(* Logix 5000 AddOnInstructionDefinition export; software revision 16.04 *)

TYPE AKD_Status :   // All connections to the drive ethernet module are established and data is successfully transferring.
STRUCT
   Profile_In_Progress : BOOL;   // Profile Move In Progress
   Block_In_Execution : BOOL;   // Block In Execution
   On_Target_Position : BOOL;   // On Target Position (1=Current Position Equals Last Target Position)
   General_Fault : BOOL;   // General Fault
   Current_Direction : BOOL;   // Current Motor Direction (0=Reverse, 1=Forward)
   Home_Level : BOOL;   // Level of Home Input
   Reg_Level : BOOL;   // Level of Registration Input
   Enable : BOOL;   // State of Enable Output
   Fault_Input_Fault : BOOL;   // Fault Input Active
   Fwd_Limit : BOOL;   // Forward Input Active
   Rev_Limit : BOOL;   // Reverse Input Active
   Positive_Limit : BOOL;   // Positive Software Limit Exceeded
   Negative_Limit : BOOL;   // Negative Software Limit Exceeded
   FE_Fault : BOOL;   // Following Error Fault
   Block_Fault : BOOL;   // Block Execution Fault
   Load_Complete : BOOL;   // Command Message Successfully Loaded
END_STRUCT
END_TYPE

TYPE AKD_Axis :   // Axis Data:
STRUCT
   Control : AKD_Control;   // Control bits to send to the drive
   Status : AKD_Status;   // Status bits received from the drive
   Input : AB:ETHERNET_MODULE_SINT_64Bytes:I:0;   // Data from the drive
   Output : AB:ETHERNET_MODULE_SINT_64Bytes:O:0;   // Data to the drive
   ResponseMsgType : SINT;   // Response type contained in latest IO response from drive. Used to check for errors
   CommandTimeout : INT;   // Time to allow for command response from drive. Dependent on scan rate and communicaiton rate
   PositionFeedback : DINT;   // Actual Position Value
   VelocityFeedback : DINT;   // Actual Velocity Value
END_STRUCT
END_TYPE

TYPE AKD_Control :   // Send Explicit Message
STRUCT
   Load_Data_Start_Profile : BOOL;   // Load Command Data / Start Profile Move
   Start_Block : BOOL;   // Execute Command block or block chain
   Incremental : BOOL;   // Incremental Position (0=Absolute, 1=Incremental)
   Direction : BOOL;   // Direction in Velocity Mode (0=Reverse, 1=Forward)
   Smooth_Stop : BOOL;   // Smooth / Controlled Stop w/ Deceleration
   Hard_Stop : BOOL;   // Hard / Immediate Stop
   Reg_Arm : BOOL;   // Arm the Registration Input
   Enable : BOOL;   // Enable Output
END_STRUCT
END_TYPE

ADD_ON_INSTRUCTION AKD_Enable   (* revision 2.0, ExecutePrescan, ExecuteEnableInFalse *)
// Enables Drive
VAR_OUTPUT
   DN : BOOL; {visible}   // Command Successful
   ER : BOOL; {visible}   // Error
END_VAR
VAR_IN_OUT
   Axis : AKD_Axis; {required}
END_VAR
VAR
   Command_Timeout : TIMER;   // Timeout Timer
   Transition : BOOL;   // Marker to transition enable bit if required.
   Transition_Complete : BOOL;   // Flag to indicate that no further transistion is required.
END_VAR

ROUTINE EnableInFalse   (* ladder *)
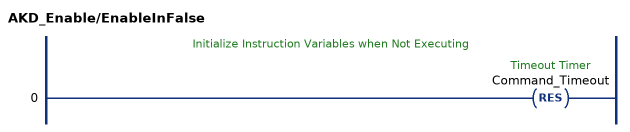
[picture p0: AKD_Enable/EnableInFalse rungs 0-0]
   // Initialize Instruction Variables when Not Executing
   0: RES(Command_Timeout);
END_ROUTINE

ROUTINE Logic   (* ladder *)
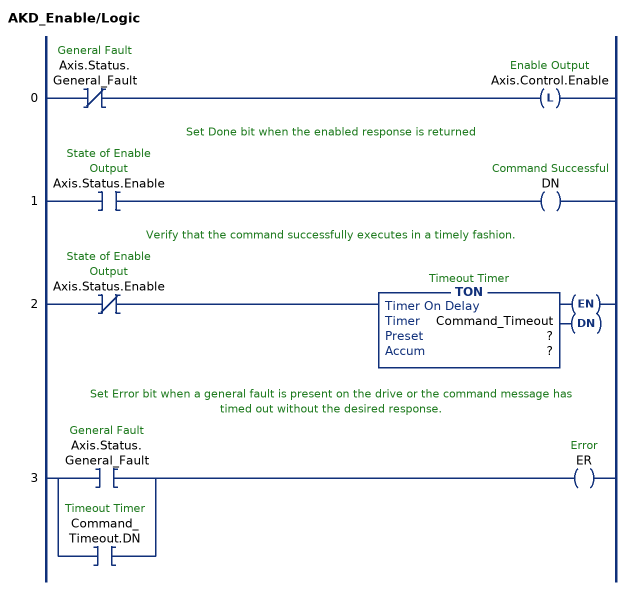
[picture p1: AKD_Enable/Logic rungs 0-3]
   0: XIO(Axis.Status.General_Fault)OTL(Axis.Control.Enable);
   // Set Done bit when the enabled response is returned
   1: XIC(Axis.Status.Enable)OTE(DN);
   // Verify that the command successfully executes in a timely fashion.
   2: XIO(Axis.Status.Enable)TON(Command_Timeout,?,?);
   // Set Error bit when a general fault is present on the drive or the command message has timed out without the desired response.
   3: [XIC(Axis.Status.General_Fault) ,XIC(Command_Timeout.DN) ]OTE(ER);
END_ROUTINE

ROUTINE Prescan   (* ladder *)
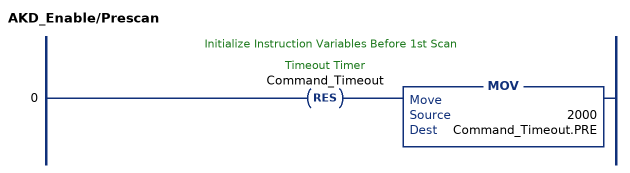
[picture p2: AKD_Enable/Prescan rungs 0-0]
   // Initialize Instruction Variables Before 1st Scan
   0: RES(Command_Timeout)MOV(2000,Command_Timeout.PRE);
END_ROUTINE
END_ADD_ON_INSTRUCTION

ADD_ON_INSTRUCTION AKD_Set_Accel   (* revision 2.1, ExecutePrescan, ExecuteEnableInFalse *)
// Set Drive Acceleration
// Revision note:
// Don't error if Command_Timeout preset is 0
VAR_OUTPUT
   DN : BOOL; {visible}   // Command Successful
   ER : BOOL; {visible}   // Error
END_VAR
VAR_IN_OUT
   Axis : AKD_Axis; {required}
END_VAR
VAR_INPUT
   Accel : DINT; {required}   // Acceleration
END_VAR
VAR
   Response_Bytes : SINT[8];
   Accel_Internal : DINT;   // Scaled Accel Value for Drive
   Command_Timeout : TIMER;   // Timeout Timer
   Command_Message_Type : SINT;   // Command Message Type
   Command_Axis_Number : SINT;   // Command Axis Number
   Response_Message_Type : SINT;   // Response Message Type
   Response_Axis_Number : SINT;   // Response Axis Number
   Command_Bytes : SINT[8];
   OS_LoadStart : BOOL;
   Step : SINT;
END_VAR

ROUTINE EnableInFalse   (* ladder *)
// EnableIn_False
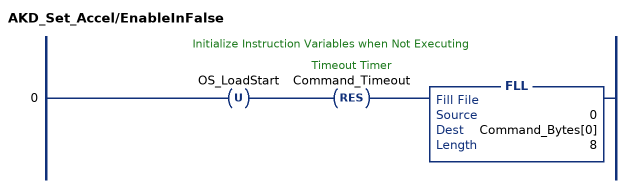
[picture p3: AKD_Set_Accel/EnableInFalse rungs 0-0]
   // Initialize Instruction Variables when Not Executing
   0: OTU(OS_LoadStart)RES(Command_Timeout)FLL(0,Command_Bytes[0],8);
END_ROUTINE

ROUTINE Logic   (* ladder *)
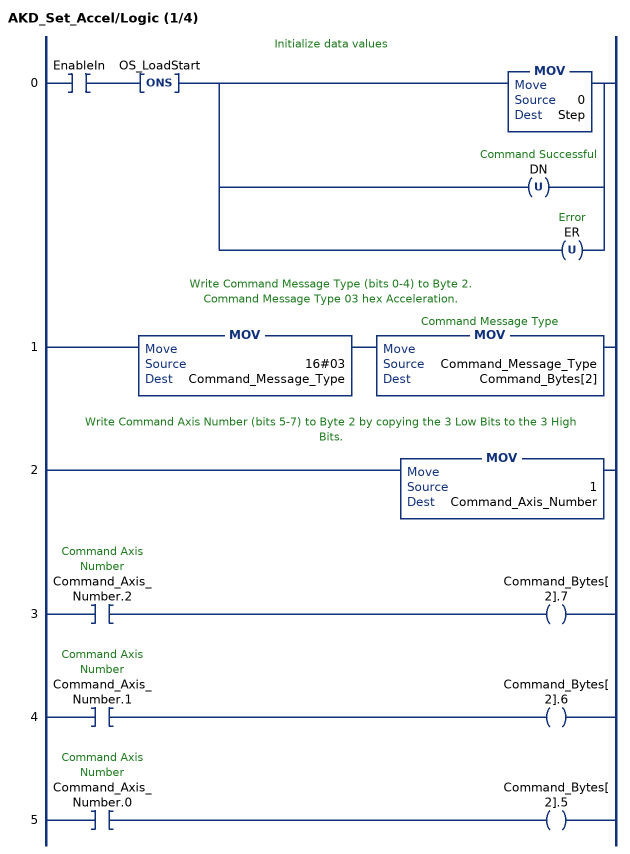
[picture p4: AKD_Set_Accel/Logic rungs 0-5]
   // Initialize data values
   0: XIC(EnableIn)ONS(OS_LoadStart)[MOV(0,Step) ,OTU(DN) ,OTU(ER) ];
   // Write Command Message Type (bits 0-4) to Byte 2.
   // Command Message Type 03 hex Acceleration.
   1: MOV(16#03,Command_Message_Type)MOV(Command_Message_Type,Command_Bytes[2]);
   // Write Command Axis Number (bits 5-7) to Byte 2 by copying the 3 Low Bits to the 3 High Bits.
   2: MOV(1,Command_Axis_Number);
   3: XIC(Command_Axis_Number.2)OTE(Command_Bytes[2].7);
   4: XIC(Command_Axis_Number.1)OTE(Command_Bytes[2].6);
   5: XIC(Command_Axis_Number.0)OTE(Command_Bytes[2].5);
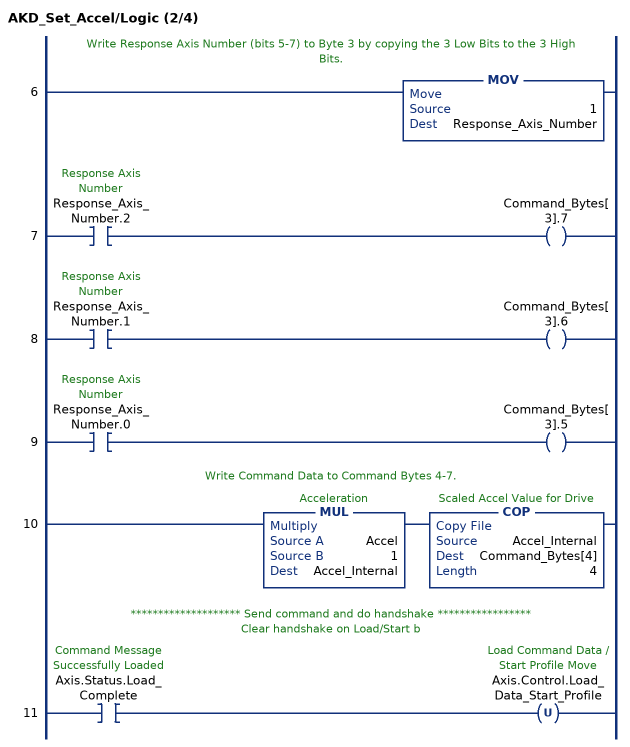
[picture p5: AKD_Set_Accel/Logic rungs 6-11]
   // Write Response Axis Number (bits 5-7) to Byte 3 by copying the 3 Low Bits to the 3 High Bits.
   6: MOV(1,Response_Axis_Number);
   7: XIC(Response_Axis_Number.2)OTE(Command_Bytes[3].7);
   8: XIC(Response_Axis_Number.1)OTE(Command_Bytes[3].6);
   9: XIC(Response_Axis_Number.0)OTE(Command_Bytes[3].5);
   // Write Command Data to Command Bytes 4-7.
   10: MUL(Accel,1,Accel_Internal)COP(Accel_Internal,Command_Bytes[4],4);
   // ******************** Send command and do handshake *****************
   // Clear handshake on Load/Start b
   11: XIC(Axis.Status.Load_Complete)OTU(Axis.Control.Load_Data_Start_Profile);
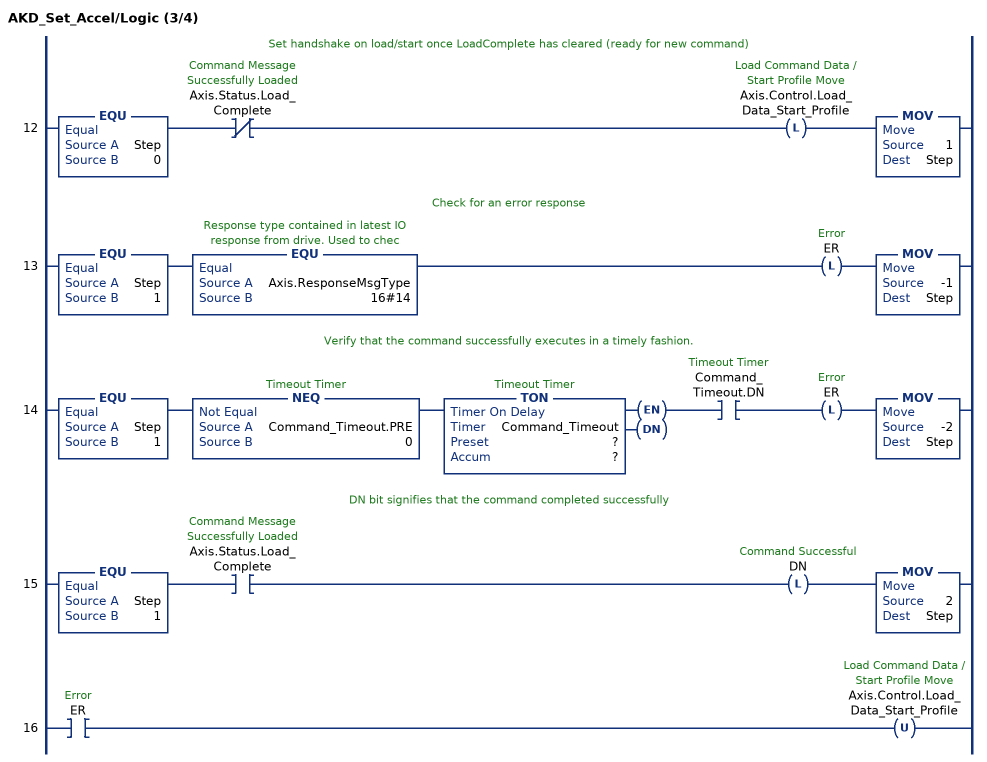
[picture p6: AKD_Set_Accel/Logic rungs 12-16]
   // Set handshake on load/start once LoadComplete has cleared (ready for new command)
   12: EQU(Step,0)XIO(Axis.Status.Load_Complete)OTL(Axis.Control.Load_Data_Start_Profile)MOV(1,Step);
   // Check for an error response
   13: EQU(Step,1)EQU(Axis.ResponseMsgType,16#14)OTL(ER)MOV(-1,Step);
   // Verify that the command successfully executes in a timely fashion.
   14: EQU(Step,1)NEQ(Command_Timeout.PRE,0)TON(Command_Timeout,?,?)XIC(Command_Timeout.DN)OTL(ER)MOV(-2,Step);
   // DN bit signifies that the command completed successfully
   15: EQU(Step,1)XIC(Axis.Status.Load_Complete)OTL(DN)MOV(2,Step);
   16: XIC(ER)OTU(Axis.Control.Load_Data_Start_Profile);
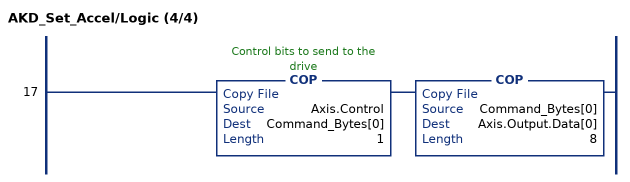
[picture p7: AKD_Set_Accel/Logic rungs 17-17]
   17: COP(Axis.Control,Command_Bytes[0],1)COP(Command_Bytes[0],Axis.Output.Data[0],8);
END_ROUTINE

ROUTINE Prescan   (* ladder *)
// Prescan
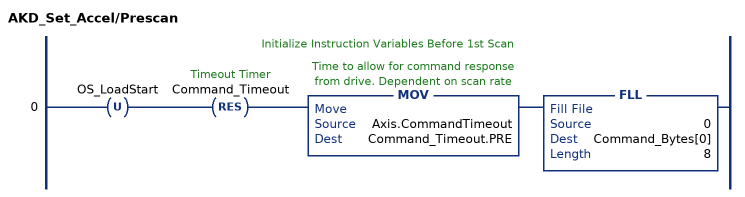
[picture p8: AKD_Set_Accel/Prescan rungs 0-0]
   // Initialize Instruction Variables Before 1st Scan
   0: OTU(OS_LoadStart)RES(Command_Timeout)MOV(Axis.CommandTimeout,Command_Timeout.PRE)FLL(0,Command_Bytes[0],8);
END_ROUTINE
END_ADD_ON_INSTRUCTION

ADD_ON_INSTRUCTION AKD_Set_Decel   (* revision 2.1, ExecutePrescan, ExecuteEnableInFalse *)
// Set Drive Deceleration
// Revision note:
// Don't error if Command_Timeout preset is 0
VAR_OUTPUT
   DN : BOOL; {visible}   // Command Successful
   ER : BOOL; {visible}   // Error
END_VAR
VAR_IN_OUT
   Axis : AKD_Axis; {required}
END_VAR
VAR_INPUT
   Decel : DINT; {required}   // Acceleration
END_VAR
VAR
   Response_Bytes : SINT[8];
   OS_LoadStart : BOOL;
   Decel_Internal : DINT;   // Scaled Decel Value for Drive
   Command_Timeout : TIMER;   // Timeout Timer
   Command_Message_Type : SINT;   // Command Message Type
   Command_Axis_Number : SINT;   // Command Axis Number
   Response_Message_Type : SINT;   // Response Message Type
   Response_Axis_Number : SINT;   // Response Axis Number
   Command_Bytes : SINT[8];
   Step : SINT;
END_VAR

ROUTINE EnableInFalse   (* ladder *)
// EnableIn_False
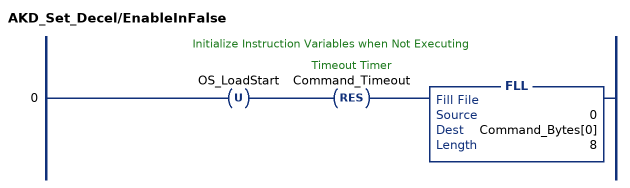
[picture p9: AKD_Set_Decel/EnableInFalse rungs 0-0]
   // Initialize Instruction Variables when Not Executing
   0: OTU(OS_LoadStart)RES(Command_Timeout)FLL(0,Command_Bytes[0],8);
END_ROUTINE

ROUTINE Logic   (* ladder *)
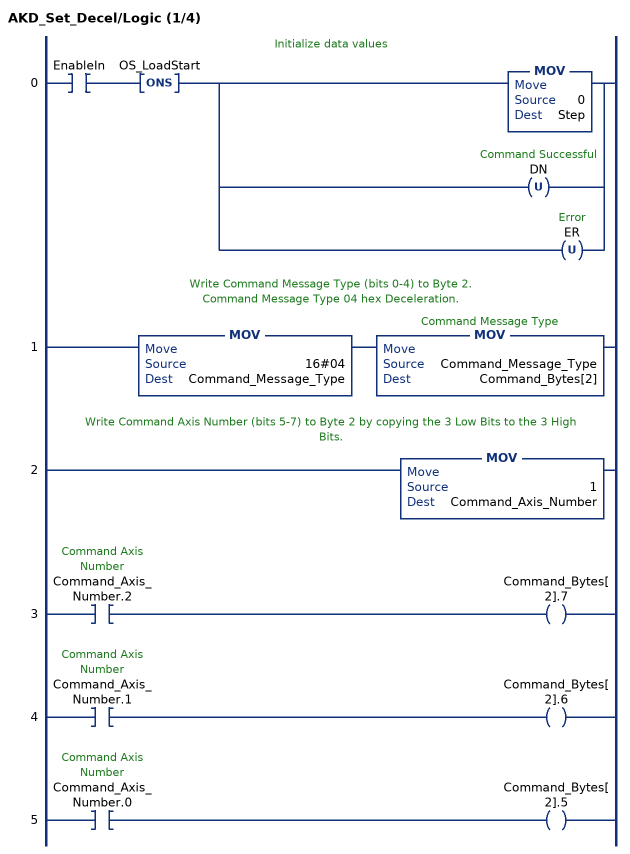
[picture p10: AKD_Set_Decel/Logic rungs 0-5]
   // Initialize data values
   0: XIC(EnableIn)ONS(OS_LoadStart)[MOV(0,Step) ,OTU(DN) ,OTU(ER) ];
   // Write Command Message Type (bits 0-4) to Byte 2.
   // Command Message Type 04 hex Deceleration.
   1: MOV(16#04,Command_Message_Type)MOV(Command_Message_Type,Command_Bytes[2]);
   // Write Command Axis Number (bits 5-7) to Byte 2 by copying the 3 Low Bits to the 3 High Bits.
   2: MOV(1,Command_Axis_Number);
   3: XIC(Command_Axis_Number.2)OTE(Command_Bytes[2].7);
   4: XIC(Command_Axis_Number.1)OTE(Command_Bytes[2].6);
   5: XIC(Command_Axis_Number.0)OTE(Command_Bytes[2].5);
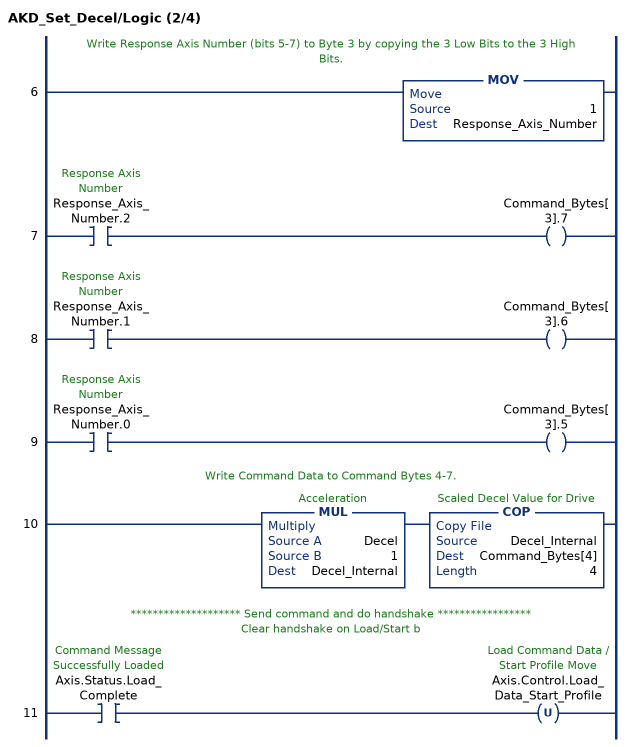
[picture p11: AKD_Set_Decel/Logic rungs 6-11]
   // Write Response Axis Number (bits 5-7) to Byte 3 by copying the 3 Low Bits to the 3 High Bits.
   6: MOV(1,Response_Axis_Number);
   7: XIC(Response_Axis_Number.2)OTE(Command_Bytes[3].7);
   8: XIC(Response_Axis_Number.1)OTE(Command_Bytes[3].6);
   9: XIC(Response_Axis_Number.0)OTE(Command_Bytes[3].5);
   // Write Command Data to Command Bytes 4-7.
   10: MUL(Decel,1,Decel_Internal)COP(Decel_Internal,Command_Bytes[4],4);
   // ******************** Send command and do handshake *****************
   // Clear handshake on Load/Start b
   11: XIC(Axis.Status.Load_Complete)OTU(Axis.Control.Load_Data_Start_Profile);
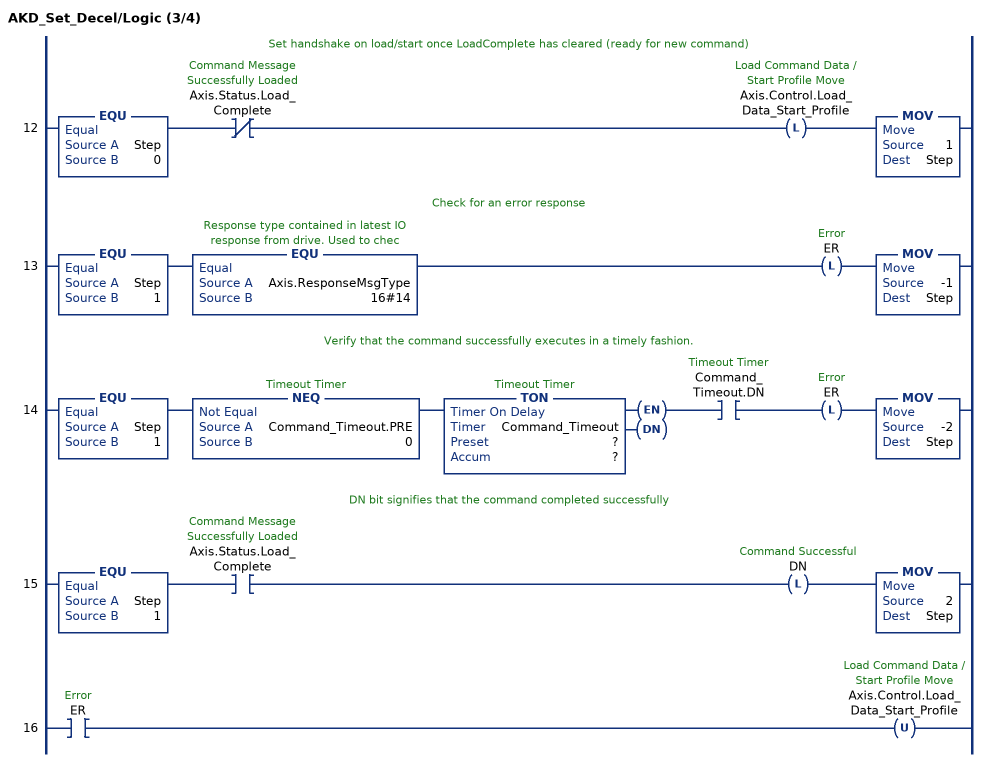
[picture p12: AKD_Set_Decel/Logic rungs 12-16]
   // Set handshake on load/start once LoadComplete has cleared (ready for new command)
   12: EQU(Step,0)XIO(Axis.Status.Load_Complete)OTL(Axis.Control.Load_Data_Start_Profile)MOV(1,Step);
   // Check for an error response
   13: EQU(Step,1)EQU(Axis.ResponseMsgType,16#14)OTL(ER)MOV(-1,Step);
   // Verify that the command successfully executes in a timely fashion.
   14: EQU(Step,1)NEQ(Command_Timeout.PRE,0)TON(Command_Timeout,?,?)XIC(Command_Timeout.DN)OTL(ER)MOV(-2,Step);
   // DN bit signifies that the command completed successfully
   15: EQU(Step,1)XIC(Axis.Status.Load_Complete)OTL(DN)MOV(2,Step);
   16: XIC(ER)OTU(Axis.Control.Load_Data_Start_Profile);
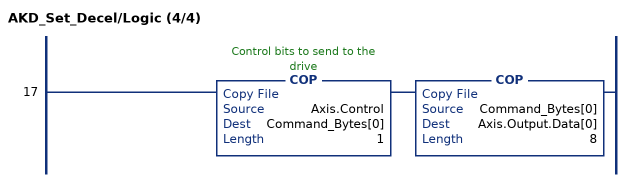
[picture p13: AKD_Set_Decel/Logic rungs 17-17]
   17: COP(Axis.Control,Command_Bytes[0],1)COP(Command_Bytes[0],Axis.Output.Data[0],8);
END_ROUTINE

ROUTINE Prescan   (* ladder *)
// Prescan
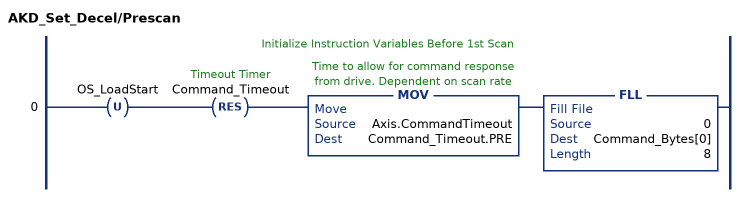
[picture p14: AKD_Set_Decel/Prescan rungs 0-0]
   // Initialize Instruction Variables Before 1st Scan
   0: OTU(OS_LoadStart)RES(Command_Timeout)MOV(Axis.CommandTimeout,Command_Timeout.PRE)FLL(0,Command_Bytes[0],8);
END_ROUTINE
END_ADD_ON_INSTRUCTION

ADD_ON_INSTRUCTION AKD_Set_Velocity   (* revision 2.1, ExecutePrescan, ExecuteEnableInFalse *)
// Set Drive Velocity
// Revision note:
// Don't error if Command_Timeout preset is 0
VAR_OUTPUT
   DN : BOOL; {visible}   // Command Successful
   ER : BOOL; {visible}   // Error
END_VAR
VAR_IN_OUT
   Axis : AKD_Axis; {required}
END_VAR
VAR_INPUT
   Velocity : DINT; {required}   // Velocity
END_VAR
VAR
   Response_Bytes : SINT[8];
   OS_LoadStart : BOOL;
   Velocity_Internal : DINT;   // Scaled Velocity Value for Drive
   Command_Timeout : TIMER;   // Timeout Timer
   Command_Message_Type : SINT;   // Command Message Type
   Command_Axis_Number : SINT;   // Command Axis Number
   Response_Message_Type : SINT;   // Response Message Type
   Response_Axis_Number : SINT;   // Response Axis Number
   Command_Bytes : SINT[8];
   Step : SINT;
END_VAR

ROUTINE EnableInFalse   (* ladder *)
// EnableIn_False
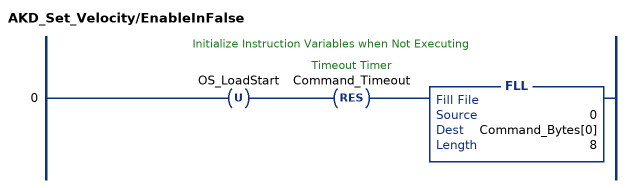
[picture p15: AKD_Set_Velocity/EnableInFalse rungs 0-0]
   // Initialize Instruction Variables when Not Executing
   0: OTU(OS_LoadStart)RES(Command_Timeout)FLL(0,Command_Bytes[0],8);
END_ROUTINE

ROUTINE Logic   (* ladder *)
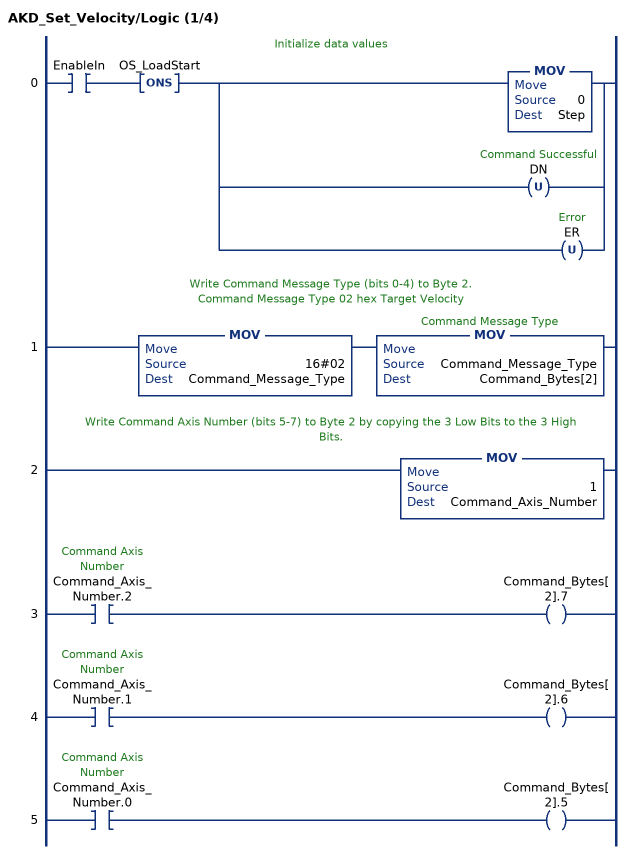
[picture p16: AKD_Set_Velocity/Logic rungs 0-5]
   // Initialize data values
   0: XIC(EnableIn)ONS(OS_LoadStart)[MOV(0,Step) ,OTU(DN) ,OTU(ER) ];
   // Write Command Message Type (bits 0-4) to Byte 2.
   // Command Message Type 02 hex Target Velocity
   1: MOV(16#02,Command_Message_Type)MOV(Command_Message_Type,Command_Bytes[2]);
   // Write Command Axis Number (bits 5-7) to Byte 2 by copying the 3 Low Bits to the 3 High Bits.
   2: MOV(1,Command_Axis_Number);
   3: XIC(Command_Axis_Number.2)OTE(Command_Bytes[2].7);
   4: XIC(Command_Axis_Number.1)OTE(Command_Bytes[2].6);
   5: XIC(Command_Axis_Number.0)OTE(Command_Bytes[2].5);
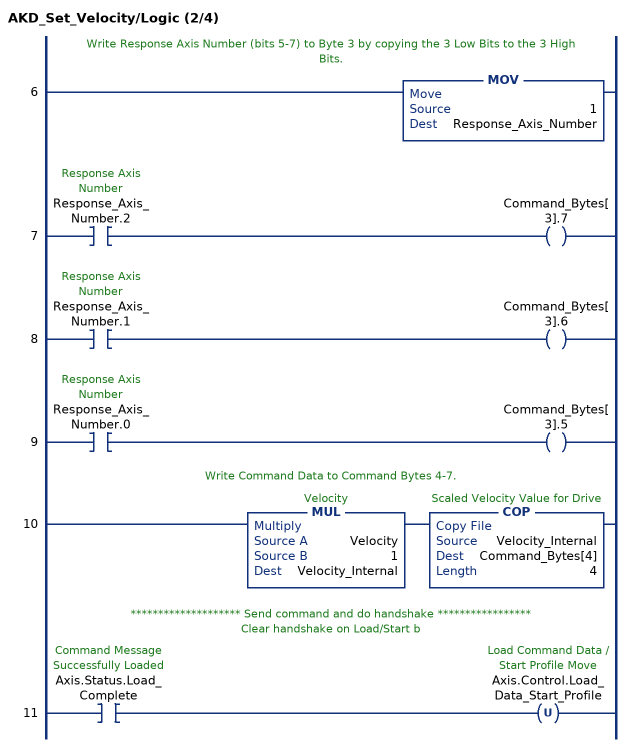
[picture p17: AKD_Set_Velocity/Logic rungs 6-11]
   // Write Response Axis Number (bits 5-7) to Byte 3 by copying the 3 Low Bits to the 3 High Bits.
   6: MOV(1,Response_Axis_Number);
   7: XIC(Response_Axis_Number.2)OTE(Command_Bytes[3].7);
   8: XIC(Response_Axis_Number.1)OTE(Command_Bytes[3].6);
   9: XIC(Response_Axis_Number.0)OTE(Command_Bytes[3].5);
   // Write Command Data to Command Bytes 4-7.
   10: MUL(Velocity,1,Velocity_Internal)COP(Velocity_Internal,Command_Bytes[4],4);
   // ******************** Send command and do handshake *****************
   // Clear handshake on Load/Start b
   11: XIC(Axis.Status.Load_Complete)OTU(Axis.Control.Load_Data_Start_Profile);
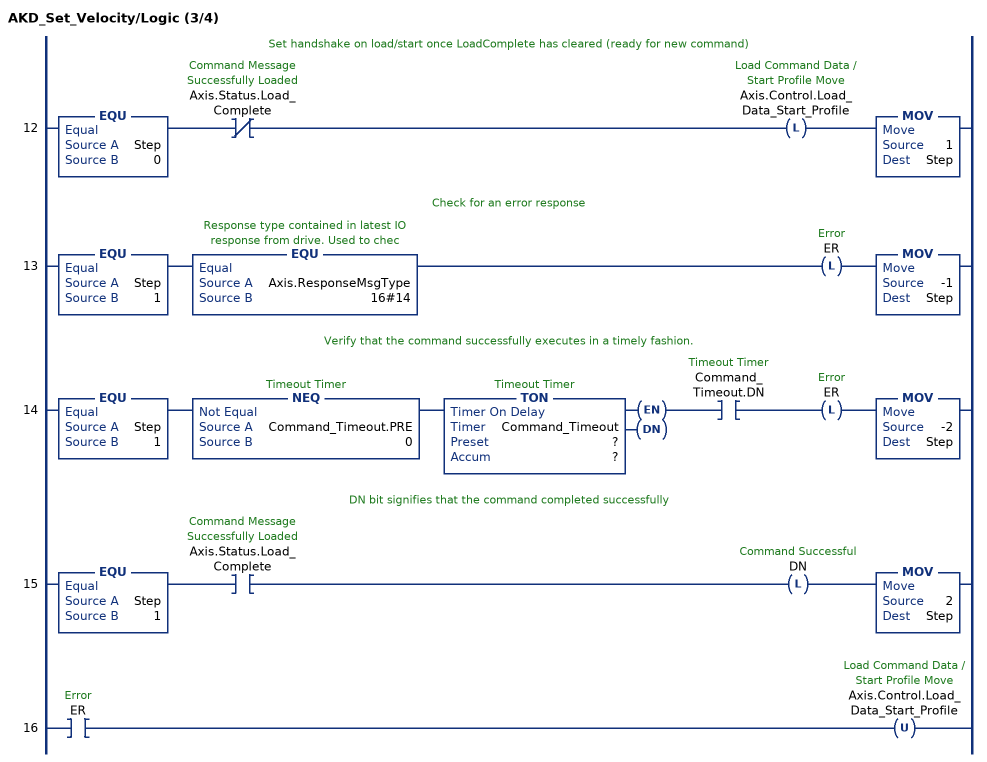
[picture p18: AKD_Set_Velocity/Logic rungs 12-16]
   // Set handshake on load/start once LoadComplete has cleared (ready for new command)
   12: EQU(Step,0)XIO(Axis.Status.Load_Complete)OTL(Axis.Control.Load_Data_Start_Profile)MOV(1,Step);
   // Check for an error response
   13: EQU(Step,1)EQU(Axis.ResponseMsgType,16#14)OTL(ER)MOV(-1,Step);
   // Verify that the command successfully executes in a timely fashion.
   14: EQU(Step,1)NEQ(Command_Timeout.PRE,0)TON(Command_Timeout,?,?)XIC(Command_Timeout.DN)OTL(ER)MOV(-2,Step);
   // DN bit signifies that the command completed successfully
   15: EQU(Step,1)XIC(Axis.Status.Load_Complete)OTL(DN)MOV(2,Step);
   16: XIC(ER)OTU(Axis.Control.Load_Data_Start_Profile);
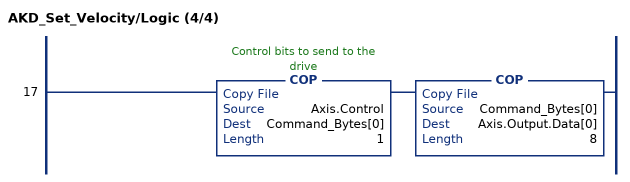
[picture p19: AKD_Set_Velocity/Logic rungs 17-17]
   17: COP(Axis.Control,Command_Bytes[0],1)COP(Command_Bytes[0],Axis.Output.Data[0],8);
END_ROUTINE
